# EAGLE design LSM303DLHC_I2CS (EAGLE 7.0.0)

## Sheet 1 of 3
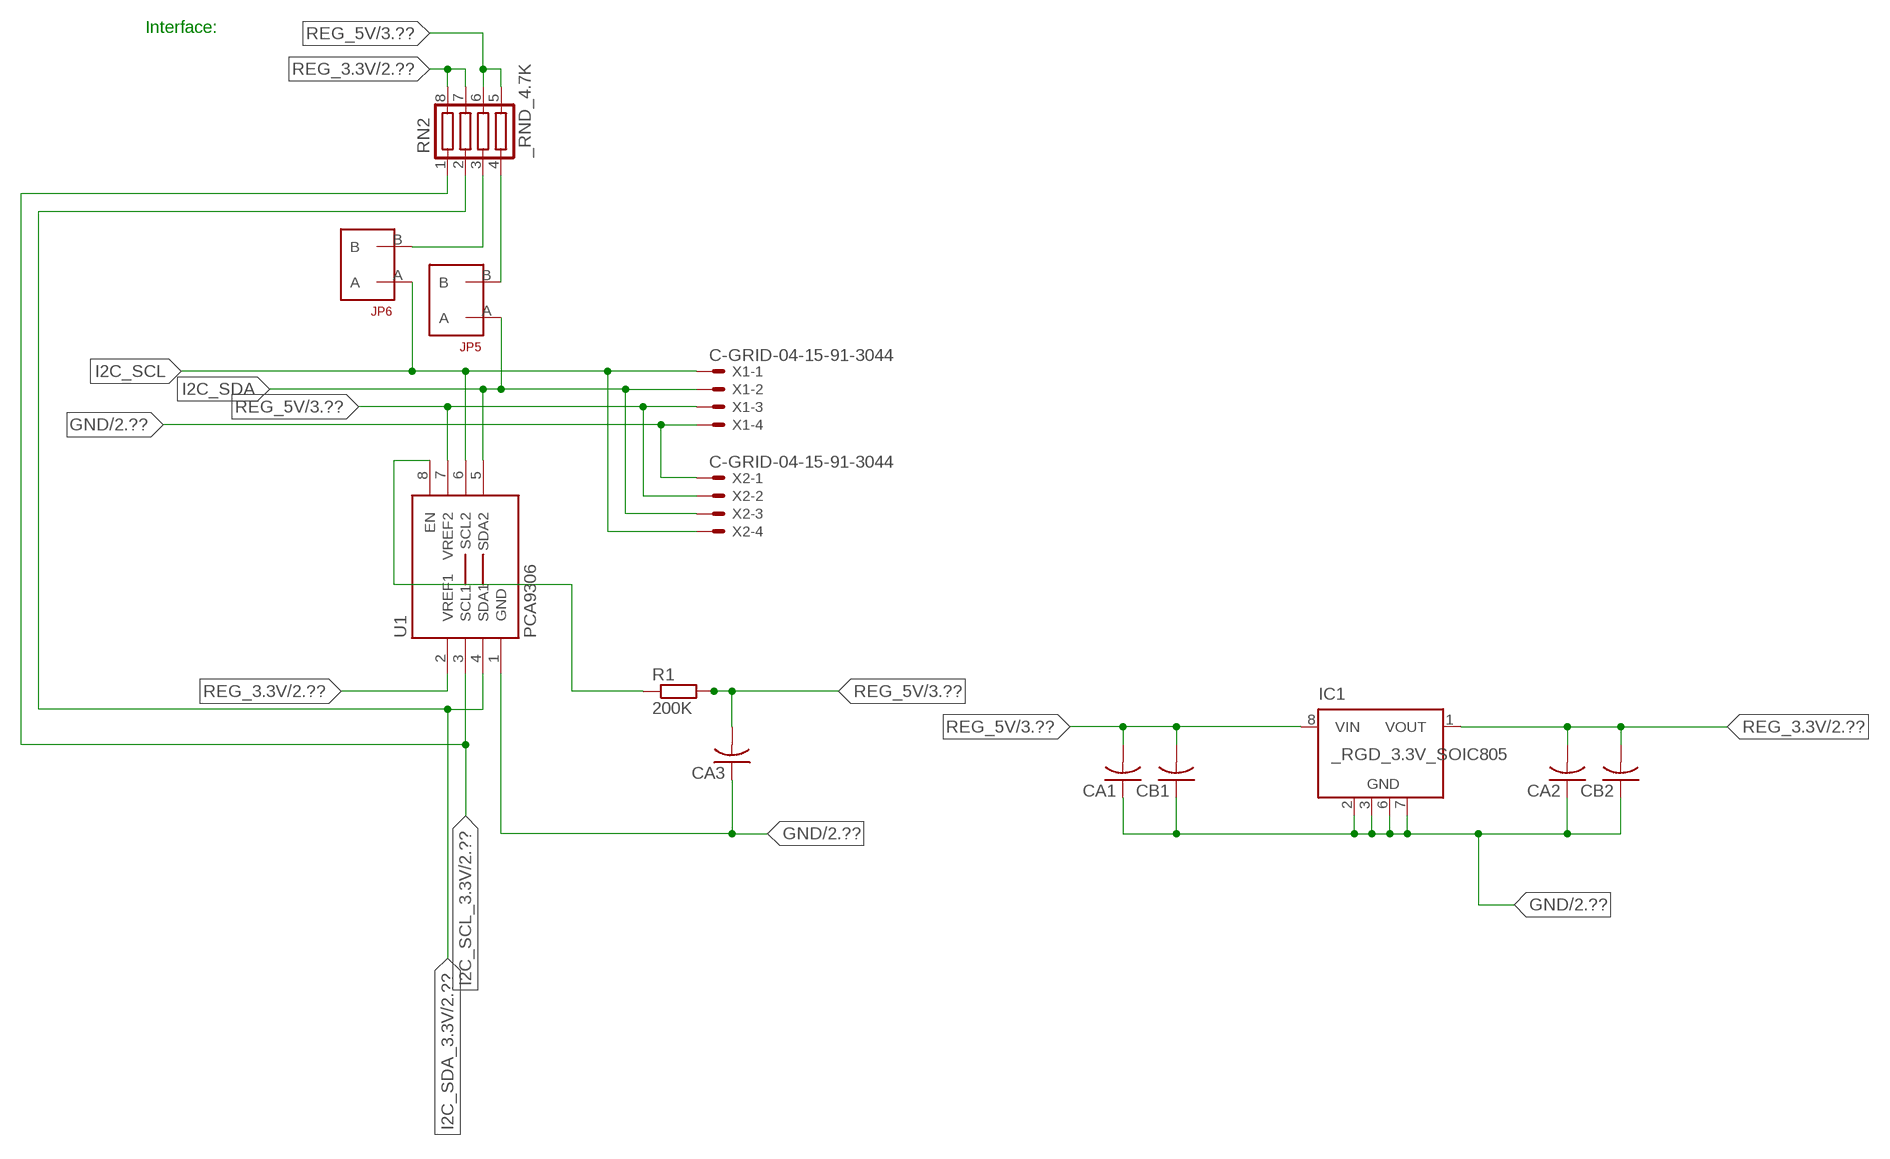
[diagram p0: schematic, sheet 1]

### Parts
CA1  CC1206KRX7R9BB104  [.1UF]
CA2  CC1206KRX7R9BB104  [.1UF]
CA3  CC1206KRX7R9BB104  [.1UF]
CB1  TMK316F106ZL-TC1206K  [TMK316F106ZL-T]
CB2  TMK316F106ZL-TC1206K  [TMK316F106ZL-T]
IC1  _RGD_3.3V_SOIC805  [_RGC_3.3V_SOIC8]
JP5  JUMPER_1X2_2MM  [JUMPER_1X2_2MM]
JP6  JUMPER_1X2_2MM  [JUMPER_1X2_2MM]
R1  200K  RESISTOR_SMT-0603  [R603]
RN2  _RND_4.7K  [RND]
U1  PCA9306  PCA9306_NCD  [PSOP-8]
X1  C-GRID-04-15-91-3044  [15-91-04]
X2  C-GRID-04-15-91-3044  [15-91-04]

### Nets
GND: CA1.1 CA2.1 CA3.1 CB1.1 CB2.1 IC1.2(GND) IC1.3(GND) IC1.6(GND) IC1.7(GND) U1.1(GND) X1.4 X2.1 ; also sheet 2,3
I2C_SCL: JP6.A U1.6(SCL2) X1.1 X2.4
I2C_SCL_3.3V: RN2.1 U1.3(SCL1) ; also sheet 2
I2C_SDA: JP5.A U1.5(SDA2) X1.2 X2.3
I2C_SDA_3.3V: RN2.2 U1.4(SDA1) ; also sheet 2
N$1: JP6.B RN2.3
N$2: JP5.B RN2.4
N$3: R1.1 U1.8(EN)
REG_3.3V: CA2.2 CB2.2 IC1.1(VOUT) RN2.7 RN2.8 U1.2(VREF1) ; also sheet 2
REG_5V: CA1.2 CA3.2 CB1.2 IC1.8(VIN) R1.2 RN2.5 RN2.6 U1.7(VREF2) X1.3 X2.2 ; also sheet 3
Unconnected: IC1.4(NC) IC1.5(NC)

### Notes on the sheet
- Interface:

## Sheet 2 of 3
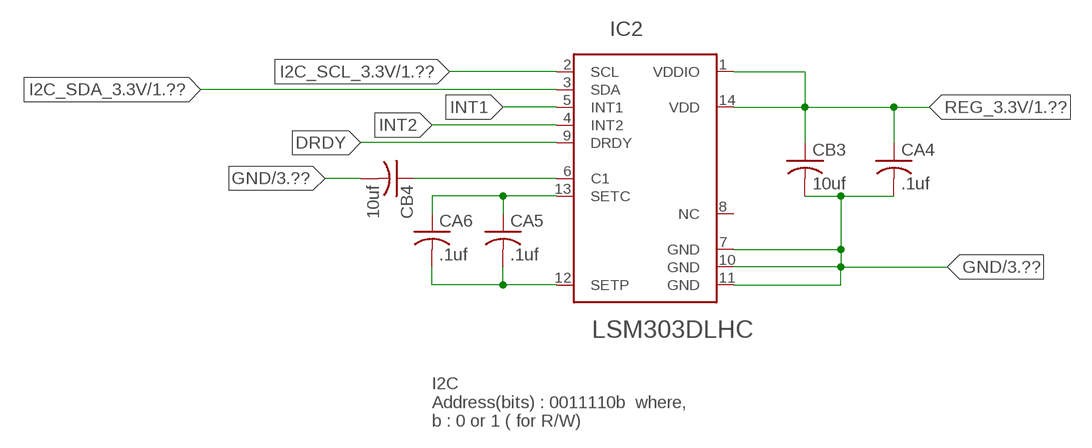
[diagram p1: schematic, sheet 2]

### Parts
CA4  .1uf  _CA_.10UF_50VC1206K  [_CA_.1UF_50V]
CA5  .1uf  _CA_.10UF_50VC1206K  [_CA_.1UF_50V]
CA6  .1uf  _CA_.10UF_50VC1206K  [_CA_.1UF_50V]
CB3  10uf  _CB_10UF_25VC1206K  [_CB_10UF_25V]
CB4  10uf  _CB_10UF_25VC1206K  [_CB_10UF_25V]
IC2  LSM303DLHC  [LGA14]

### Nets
DRDY: IC2.9(DRDY)
GND: CA4.2 CB3.2 CB4.2 IC2.7(GND) IC2.10(GND) IC2.11(GND) ; also sheet 1,3
I2C_SCL_3.3V: IC2.2(SCL) ; also sheet 1
I2C_SDA_3.3V: IC2.3(SDA) ; also sheet 1
INT1: IC2.5(INT1)
INT2: IC2.4(INT2)
N$4: CB4.1 IC2.6(C1)
N$5: CA5.1 CA6.1 IC2.13(SETC)
N$6: CA5.2 CA6.2 IC2.12(SETP)
REG_3.3V: CA4.1 CB3.1 IC2.1(VDDIO) IC2.14(VDD) ; also sheet 1
Unconnected: IC2.8(NC)

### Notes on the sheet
- I2C 
  Address(bits) : 0011110b  where,
  b : 0 or 1 ( for R/W)

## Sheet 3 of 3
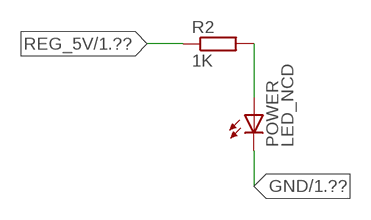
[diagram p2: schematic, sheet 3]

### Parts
POWER  LED_NCD  [CHIPLED_0603]
R2  1K  RESISTOR_SMT-0402  [R402]

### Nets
GND: POWER.C ; also sheet 1,2
N$7: POWER.A R2.2
REG_5V: R2.1 ; also sheet 1

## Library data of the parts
CA1-CA3 = NCD_ULTIMATE_LIBRARY:CC1206KRX7R9BB104: Capacitor CA .1uF 50V SMT C1206K CC1206KRX7R9BB104
CA4-CA6 = NCD_ULTIMATE_LIBRARY:_CA_.10UF_50V: Capacitor .1uF SMT
CB1 CB2 = NCD_ULTIMATE_LIBRARY:TMK316F106ZL-T: Capacitor CB 10uF SMT 1206 TMK316F106ZL-T
CB3 CB4 = NCD_ULTIMATE_LIBRARY:_CB_10UF_25V: Capacitor 10uF SMT
IC1 = NCD_ULTIMATE_LIBRARY:_RGD_3.3V_SOIC8: Regulator Linear 3.3V Chip Positive VOLTAGE REGULATOR Digikey 497-1199-2-ND/L78L33ACD13TR
IC2 = NCD_ULTIMATE_ROHIT:LSM303DLHC
JP5 JP6 = NCD_ULTIMATE_CONNECTORS:JUMPER_1X2_2MM
POWER = NCD_ULTIMATE_LIBRARY:LED_NCD: LED Digikey 754-1132-2-ND/APT2012SRCPRV
R1 R2 = NCD_ULTIMATE_LIBRARY:RESISTOR_SMT: NCD Resistor
RN2 = NCD_ULTIMATE_LIBRARY:_RND_4.7K: Resistor Array RND SMT 4.7K x 4 Single Resistor Source: http://www.ctscorp.com/components/Datasheets/CTSChipArrayDs.pdf Digikey 742C083472JPTR-ND/742C083472JP; OC_FARNELL: unknown; OC_NEWARK: unknown
U1 = NCD_ULTIMATE_LIBRARY:PCA9306_NCD: NCD Bidirectional I2C level shifter. NOT compatible with all available part number pinout schemes- DOUBLE CHECK!!!; PROD_ID: IC-10023
X1 X2 = NCD_ULTIMATE_CONNECTORS:C-GRID-04: CONNECTOR 4-Pos I2C wire to board 2.54 mm (0.100") pitch header Digikey WM1342-ND/0015912045; OC_FARNELL: unknown; OC_NEWARK: unknown

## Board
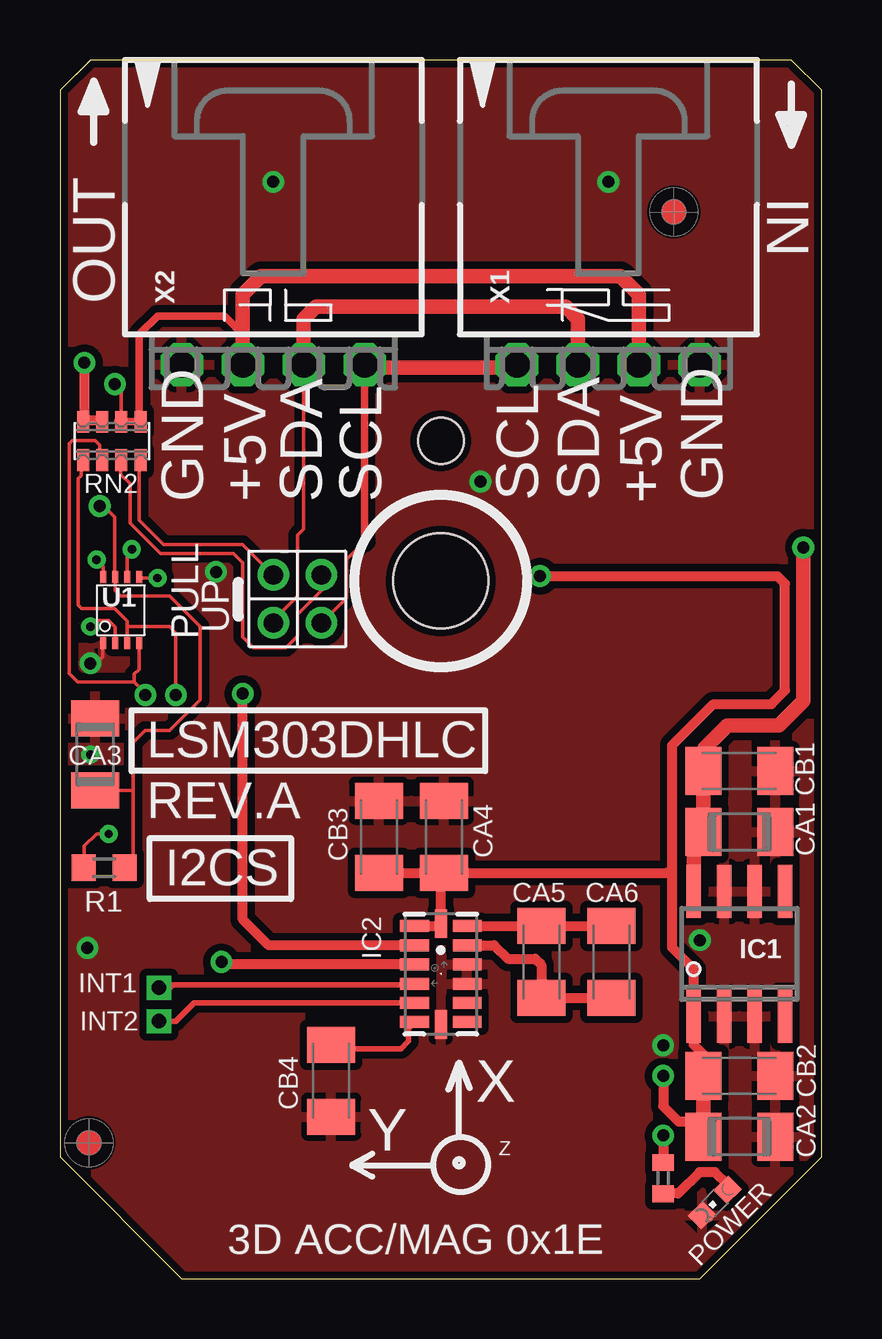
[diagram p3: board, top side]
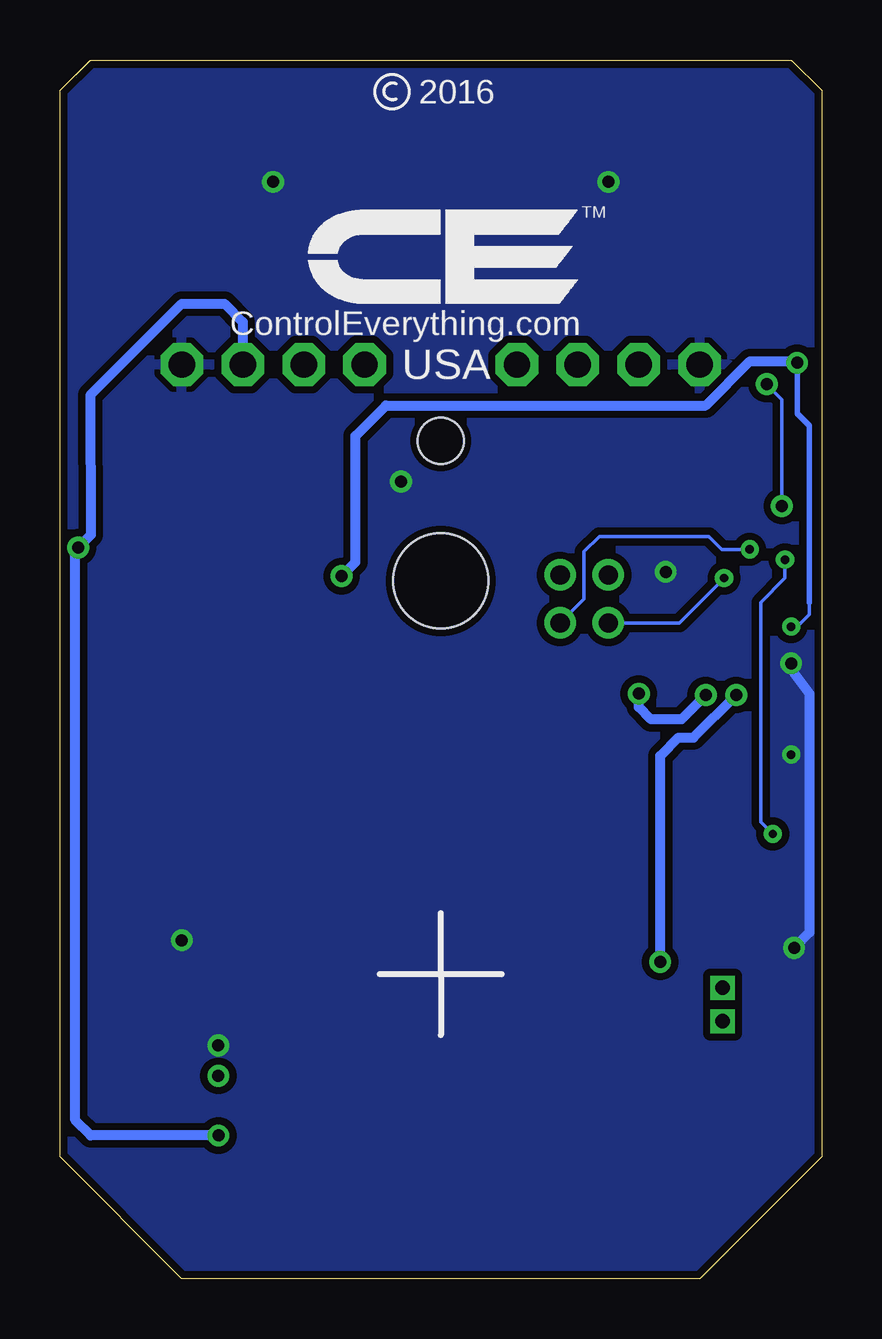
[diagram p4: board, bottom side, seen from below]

Size 31.75 x 50.8 mm. Coordinates in mm from the lower left corner, seen from the top.
Outline: 32 segments
Copper layers (1*16): Top 0.035mm / dielectric 1.5mm / Bottom 0.035mm
Design rules "default": minimum track width 5mil, minimum drill 24mil, track to track 5mil, track to pad 5mil, pad to pad 5mil, via to via 5mil, smd to smd 5mil, copper to edge 10mil, drill to drill 8mil, minimum pad ring 10mil, minimum via ring 8mil, stop-mask expansion 2mil, vias tented up to drill 0mil, thermal gap 10mil
Holes 3.96 mm at 15.88,29.08
Holes 1.91 mm at 15.88,34.93

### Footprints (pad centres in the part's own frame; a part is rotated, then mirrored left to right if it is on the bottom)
.1UF = smd 1.5 x 2: 1 -1.5,0; 2 1.5,0
_CA_.1UF_50V = smd 1.5 x 2: 1 -1.5,0; 2 1.5,0
TMK316F106ZL-T = smd 1.5 x 2: 1 -1.5,0; 2 1.5,0
_CB_10UF_25V = smd 1.5 x 2: 1 -1.5,0; 2 1.5,0
_RGC_3.3V_SOIC8 = smd 0.6 x 2.2: 1 -1.905,-2.6; 2 -0.635,-2.6; 3 0.635,-2.6; 4 1.905,-2.6; 5 1.905,2.6; 6 0.635,2.6; 7 -0.635,2.6; 8 -1.905,2.6
LGA14 = smd 0.5 x 1.2: 1 2,1.1; 2 1.2,1.1; 3 0.4,1.1; 4 -0.4,1.1; 5 -1.2,1.1; 6 -2,1.1; 8 -2,-1.1; 9 -1.2,-1.1; 10 -0.4,-1.1; 11 0.4,-1.1; 12 1.2,-1.1; 13 2,-1.1 | smd 1.2 x 0.5: 7 -2.1,0; 14 2.1,0
JUMPER_1X2_2MM = drill 0.8: A 0,2; B 0,0
CHIPLED_0603 = smd 0.8 x 0.876: A 0,-0.75; C 0,0.75
R603 = smd 1 x 1.1: 1 -0.85,0; 2 0.85,0
R402 = smd 0.7 x 0.9: 1 -0.65,0; 2 0.65,0
RND = smd 0.5 x 0.9: 1 -1.2,-0.8; 2 -0.4,-0.8; 3 0.4,-0.8; 4 1.2,-0.8; 5 1.2,0.8; 6 0.4,0.8; 7 -0.4,0.8; 8 -1.2,0.8
PSOP-8 = smd 0.25 x 0.5: 1 -0.73,-1.37; 2 -0.23,-1.37; 3 0.27,-1.37; 4 0.77,-1.37; 5 0.77,1.38; 6 0.27,1.38; 7 -0.23,1.38; 8 -0.73,1.38
15-91-04 = drill 1.1 pad 1.778 octagon: 1 -3.81,-7.62; 2 -1.27,-7.62; 3 1.27,-7.62; 4 3.81,-7.62

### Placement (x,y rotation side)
CA1  28.32,18.62 180 top
CA2  28.32,5.92 180 top
CA3  1.46,21.86 270 top
CA4  16,18.42 90 top
CA5  20.07,13.21 270 top
CA6  22.99,13.21 270 top
CB1  28.32,21.16 180 top
CB2  28.32,8.46 180 top
CB3  13.3,18.42 90 top
CB4  11.3,8.26 270 top
IC1  28.32,13.54 0 top
IC2  15.88,12.7 90 top
JP5  8.89,29.34 180 top
JP6  10.9,29.34 180 top
POWER  27.3,3.18 135 top
R1  1.84,17.13 0 top
R2  25.15,4.19 270 top
RN2  2.16,34.93 0 top
U1  2.54,27.86 0 top
U$5  [VISION_REF10]  1.21,5.66 90 top
U$28  [VISION_REF10]  25.59,44.46 90 top
X1  22.86,45.72 0 top
X2  8.89,45.72 0 top

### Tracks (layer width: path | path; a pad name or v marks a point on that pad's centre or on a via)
GND  (via drill 0.35, 0.5)
  Top 0.152: CA3.1 1.52,23.42 1.52,23.62 | U1.1 1.78,26.46 1.78,25.91 1.52,25.65 v1.27,25.65
  Bottom 0.406: v1.27,25.65 1.27,25.4 0.51,24.38 0.51,14.43 v1.15,13.79
  other vias: 8.89,45.72 22.86,45.72 25.15,9.73 17.53,33.22 26.67,14.11 6.5,29.46 1.27,21.84
  pour Bottom (isolate 0.305): -0.64,5.08 -0.64,49.53 1.27,51.44 30.48,51.44 32.38,49.53 32.38,5.08 26.67,-0.63 5.08,-0.63
  pour Top (isolate 0.305): 4.45,-1.27 -1.27,4.45 -1.27,50.17 0.64,52.07 31.11,52.07 33.02,50.17 33.02,4.45 27.3,-1.27
I2C_SCL  (via drill 0.35)
  Top 0.152: 12.7,30.73 11.94,29.97 11.94,28.38 JP6.A | v3,30.4 2.81,30.47 U1.6
  Top 0.305: 12.7,30.73 X2.4
  Top 0.406: X2.4 12.7,37.97 | 19.05,37.97 X1.1
  Top 0.61: 12.7,37.97 19.05,37.97
  Bottom 0.152: JP6.A 9.91,28.33 9.91,30.3 9.27,30.94 4.7,30.94 4.17,30.4 v3,30.4
I2C_SCL_3.3V  (via drill 0.5)
  Top 0.152: RN2.1 0.89,34.07 0.89,33.48 0.77,33.35 0.77,28.08 0.9,27.94 2.29,27.94 2.81,27.42 2.81,27.18 | 2.81,27.18 U1.3 | v4.83,24.33 v4.83,24.34 4.83,26.92 4.57,27.18 2.81,27.18
  Top 0.406: IC2.2 8.71,13.9 7.62,14.99 v7.62,24.38
  Bottom 0.406: v4.83,24.33 5.84,23.32 7.11,23.32 7.62,23.83 v7.62,24.38
I2C_SDA  (via drill 0.35)
  Top 0.152: JP5.A 8.89,27.44 9.91,28.45 9.91,30.99 10.16,31.24 10.16,34.92 X2.3 | U1.5 3.34,29.21 v4.06,29.21
  Top 0.61: X2.3 10.16,40.01 10.67,40.51 21.09,40.51 21.59,40.01 X1.2
  Bottom 0.152: v4.06,29.21 5.94,27.34 JP5.A
I2C_SDA_3.3V  (via drill 0.5)
  Top 0.152: RN2.2 1.65,34.14 1.65,34.75 1.46,34.94 0.51,34.94 0.38,34.81 0.38,27.89 0.38,25.22 0.74,24.87 3.1,24.87 | 3.1,24.87 3.56,24.41 v3.56,24.33 | U1.4 3.3,25.4 3.1,25.2 3.1,24.87
  Top 0.406: IC2.3 6.73,13.1 v6.73,13.21
  Bottom 0.406: v3.56,24.33 5.34,22.56 5.97,22.56 6.73,21.79 v6.73,13.21
INT1  (via drill 0.6)
  Top 0.229: IC2.5 14.77,11.49 5.59,11.49 4.83,10.73 v4.13,10.73
INT2  (via drill 0.6)
  Top 0.229: IC2.4 14.73,12.26 4.7,12.26 4.57,12.13 v4.13,12.13
N$1
  Top 0.152: JP6.B 10.92,29.31 10.92,28.7 9.91,27.69 9.91,26.8 9.42,26.31 8.06,26.31 7.62,26.75 7.62,29.84 7.24,30.23 4.19,30.23 2.92,31.5 2.92,33.15 2.54,33.53 2.54,34.1 RN2.3
  Top 0.305: 2.54,34.02 RN2.3
N$2
  Top 0.152: JP5.B 7.62,30.61 4.32,30.61 3.3,31.62 3.3,34.07 RN2.4
  Top 0.305: 3.37,33.88 RN2.4
N$3  (via drill 0.35)
  Top 0.152: R1.1 1.02,17.16 1.02,18.03 1.52,18.54 v2.03,18.54 | v1.52,29.97 1.81,29.69 U1.8
  Bottom 0.152: v2.03,18.54 2.54,19.05 2.54,28.19 1.52,29.21 v1.52,29.97
N$4
  Top 0.229: IC2.6 14.54,10.47 14.54,9.91 14.22,9.59 12.26,9.59 12.09,9.76 CB4.1
N$5
  Top 0.406: IC2.13 CA5.1 CA6.1
N$6
  Top 0.406: IC2.12 18.1,13.9 18.67,13.34 19.81,13.34 20.07,13.08 CA5.2 CA6.2
N$7
  Top 0.406: POWER.A 27.84,3.92 27.3,4.45 26.67,4.45 25.78,3.56 25.16,3.56 R2.2
REG_3.3V  (via drill 0.35, 0.5)
  Top 0.152: v1.27,27.18 1.52,27.43 2.03,27.43 2.31,27.16 U1.2
  Top 0.406: CB2.2 26.82,9.35 26.42,9.75 26.42,10.36 | v25.15,8.46 25.15,7.19 25.78,6.55 26.82,6.55 | IC1.1 26.42,12.9 25.53,13.79 25.53,17.08 | 25.53,17.08 25.53,22.24 27.24,23.95 29.66,23.95 30.23,24.52 30.23,28.97 29.91,29.29 v20.02,29.29 | 26.52,5.62 CA2.2 | v1.02,38.18 1.02,35.78 | 1.02,35.78 RN2.8 | 1.02,35.78 1.71,35.78 RN2.7 | IC2.1 15.78,14.7 IC2.14 15.88,17.42 CA4.1 | 15.84,16.7 CA4.1 | CA4.1 25.3,16.92 25.53,17.08 | CB3.1 CA4.1
  Top 0.61: CB2.2 26.82,6.55 CA2.2 | 26.42,10.36 IC1.1
  Bottom 0.152: 0.51,28.19 0.51,27.69 1.02,27.18 v1.27,27.18
  Bottom 0.229: 0.51,28.19 0.51,35.56 1.02,36.07 v1.02,38.18
  Bottom 0.406: v1.02,38.18 1.08,38.24 2.99,38.24 4.83,36.4 18.16,36.4 19.43,35.13 19.43,29.87 19.94,29.34 19.96,29.34 v20.02,29.29
REG_5V  (via drill 0.5)
  Top 0.152: RN2.6 2.56,37.01 v2.29,37.29 | R1.2 3.05,17.49 3.05,20.36 | 3.05,20.36 3.05,22.35 3.56,22.86 4.57,22.86 5.84,24.13 5.84,27.18 4.57,28.45 2.54,28.45 2.31,28.68 U1.7 2.29,29.27 2.29,31.75 1.83,32.21 v1.65,32.21 | CA3.2 3.05,20.36
  Top 0.305: 7.62,39.37 7.5,39.37 | 2.42,35.74 RN2.6 RN2.5 3.31,35.8 3.31,39.37 4.07,40.13 6.86,40.13 7.62,39.37 | X2.2 7.62,39.37
  Top 0.406: v25.15,5.97 R2.1
  Top 0.61: X1.3 24.13,41.02 23.37,41.78 8.38,41.78 7.62,41.02 X2.2 | IC1.8 26.42,18.21 CA1.2 CB1.2 26.86,21.2 26.86,22.11 27.82,23.06 29.98,23.06 30.99,24.08 v30.99,30.48
  Bottom 0.152: v1.65,32.21 1.65,36.65 v2.29,37.29
  Bottom 0.406: v25.15,5.97 30.48,5.97 31.11,6.6 31.11,30.36 v30.99,30.48 30.47,31 30.48,36.83 26.67,40.64 24.89,40.64 24.13,39.88 24.13,38.73 | X1.3 24.13,38.23 | 24.13,38.23 24.13,38.61 24.13,38.73 | 24.13,38.73 24.13,38.74 24.13,38.23 | 24.13,38.23 X1.3 | 24.13,38.23

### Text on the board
tPlace: X | Y | Z
tNames: IN | OUT | GND | +5V | SDA | SCL | SCL | SDA | +5V | GND | PULL | UP | LSM303DHLC | REV.A | I2CS | INT1 | INT2 | 3D ACC/MAG 0x1E
bNames: 2016 | TM | ControlEverything.com | USA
